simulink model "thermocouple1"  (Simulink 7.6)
settings: Solver=ode15s  StartTime=0.0  StopTime=1  RelTol=1e-3
InitFcn:
  | clear all
  | close all
  | clc
  | fem_temp_thermocouple
libraries: nesl_utility x3, fl_lib x1

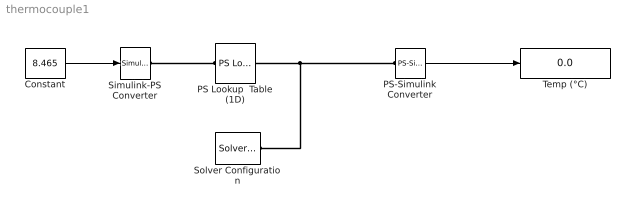
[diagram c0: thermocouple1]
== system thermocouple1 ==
  Constant : Constant  Value=8.465
  PS Lookup  Table (1D) : fl_lib/Physical Signals/Lookup Tables/PS Lookup Table (1D)  DialogController=NetworkEngine.DynNeDlgSource  SystemSampleTime=-1  x_t=fem  y_t=temp  interp_method=1  extrap_method=1  dbg=0  LocalVarLogging=[]
  PS-Simulink Converter : nesl_utility/PS-Simulink Converter  DialogController=NetworkEngine.DynNeUtilDlgSource  SystemSampleTime=-1  PhysicalDomain=network_engine_domain  LeftPortType=input  RightPortType=output  SubClassName=ps_output  Unit=1  AffineConversion=off
  Simulink-PS Converter : nesl_utility/Simulink-PS Converter  DialogController=NetworkEngine.DynNeUtilDlgSource  SystemSampleTime=-1  PhysicalDomain=network_engine_domain  LeftPortType=input  RightPortType=output  SubClassName=ps_input  Unit=1  AffineConversion=off  InputFilterTimeConstant=.001  UdotUserProvided=0
  Solver Configuration : nesl_utility/Solver Configuration  DialogController=NetworkEngine.DynNeUtilDlgSource  SystemSampleTime=-1  PhysicalDomain=network_engine_domain  LeftPortType=input  RightPortType=generic  SubClassName=solver  Accelerate=off  Profile=off  ResidualTolerance=1e-9  MaxNonlinIter=3  MaxModeIter=2  DoFixedCost=off  UseLocalSampling=off  DoDC=off  LinearAlgebra=Sparse  LocalSolverSampleTime=.001  LocalSolverChoice=NE_BACKWARD_EULER_ADVANCER  UseLocalSolver=off
  Temp (°C) : Display
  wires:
  Constant/1 -> Simulink-PS Converter/1
  PS-Simulink Converter/1 -> Temp (°C)/1
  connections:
  PS Lookup  Table (1D)/LConn1 -- Simulink-PS Converter/RConn1
  Solver Configuration/RConn1 -- PS Lookup  Table (1D)/RConn1 -- PS-Simulink Converter/LConn1
